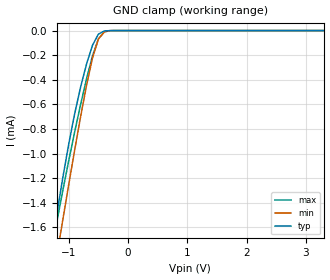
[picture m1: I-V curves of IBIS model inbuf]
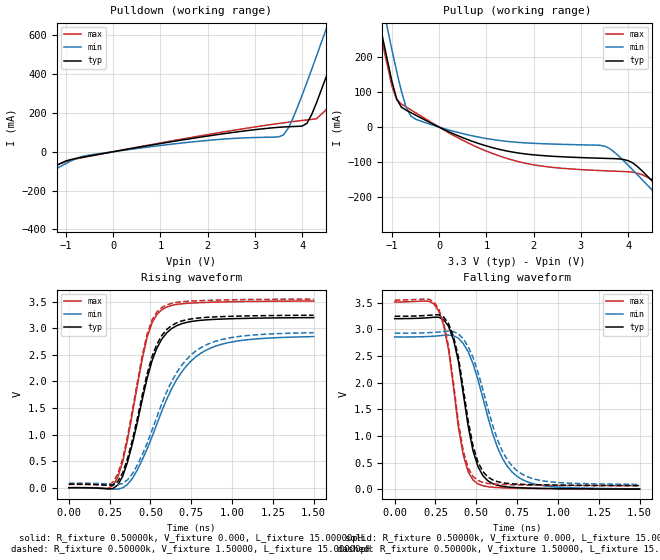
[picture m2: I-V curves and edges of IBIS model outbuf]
| IBIS file 4v38075z.ibs created by s2ibis2 version 1.2
| North Carolina State University Electronics Research Laboratory  1995
[IBIS ver]   3.2
[File name]   4v38075z.ibs
[File Rev]   0.2
[Date]   08/30/2004
[Source]   Integrated Device Technology, Inc.
[Notes]   1.Temperatures: typ=25C, min=150C, max=0C 2.Ramp rates based
   on 500 ohm load.
[Disclaimer] Integrated Device Technology, Inc. ("IDT") hereby grants the
   user of this IBIS model a non-exclusive, nontransferable
   license to use this IBIS model under the following terms. The
   user is granted this license only to use the IBIS model and is
   not granted rights to sell, copy (except as needed to run the
   IBIS model), rent, lease or sub-license the IBIS model in
   whole or in part, or in modified form to anyone. The User may
   modify the IBIS model to suit its specific applications, but
   rights to derivative works and such modifications shall belong
   to IDT. This IBIS model is provided on an AS IS" basis and IDT
   makes absolutely no warranty with respect to the information
   contained herein. IDT DISCLAIMS AND CUSTOMER WAIVES ALL
   WARRANTIES, EXPRESS AND IMPLIED, INCLUDING WARRANTIES OF
   MERCHANTABILITY AND FITNESS FOR A PARTICULAR PURPOSE. THE
   ENTIRE RISK AS TO QUALITY AND PERFORMANCE IS WITH THE USER
   ACCORDINGLY, IN NO EVENT SHALL IDT BE LIABLE FOR ANY DIRECT OR
   INDIRECT DAMAGES, WHETHER IN CONTRACT OR TORT, INCLUDING ANY
   LOST PROFITS OR OTHER INCIDENTAL, CONSEQUENTIAL, EXEMPLARY, OR
   PUNITIVE DAMAGES ARISING OUT OF THE USE OR APPLICATION OF THE
   IBIS model. Further, IDT reserves the right to make changes
   without notice to any product herein to improve reliability,
   function, or design. IDT does not convey any license under
   patent rights or any other intellectual property rights,
   including those of third parties. IDT is not obligated to
   provide maintenance or support for the licensed IBIS model.
[Copyright]   Copyright 1997, Integrated Device Technology, Inc. all rights
   reserved
|   Component idt4v38075z
[Component]   idt4v38075z
[Manufacturer]   Integrated Device Technology, Inc.
[Package]
| variable   typ   min   max
R_pkg   53.14m   52.77m   53.55m
L_pkg   5.18nH   4.04nH   6.38nH
C_pkg   0.38pF   0.224pF   0.551pF
[Pin]  signal_name   model_name   R_pin   L_pin   C_pin
1   O5   outbuf
2   VCC   POWER
3   IN   inbuf
4   GND   GND
5   O1   outbuf
6   O2   outbuf
7   O3   outbuf
8   O4   outbuf
| Models and submodels in the file (2): inbuf (Input), outbuf (Output)
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|   Model inbuf
[Model]   inbuf
Model_type   Input
Polarity   Inverting
Vinl =  0.80000V
Vinh =  2.00000V
Vmeas =  1.50000V
C_comp   2.60000pF   NA   NA
[Temperature Range]   25.00000   0.15000k   0.000
[Voltage Range]   3.30000V   3.00000V   3.60000V
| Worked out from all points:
|   GND clamp passes 1 mA (typ) near -1.03 V on its own axis
[GND_clamp]
| voltage   I(typ)   I(min)   I(max)
-3.3V     -8.354mA   -8.197mA   -8.333mA
-1.3V     -1.792mA   -2.121mA   -1.821mA
-1.2V     -1.488mA   -1.827mA   -1.552mA
-1.1V     -1.195mA   -1.537mA   -1.299mA
-1V       -921.4uA   -1.25mA    -1.056mA
-900mV    -674.9uA   -969.9uA   -823.3uA
-800mV    -458.9uA   -699.2uA   -600.1uA
-700mV    -271.4uA   -445uA     -391uA
-600mV    -119.9uA   -223.2uA   -205.7uA
-500mV    -28.6uA    -68.61uA   -67.73uA
-400mV    -2.904uA   -10.33uA   -9.139uA
3.3V      2.359pA    530.5pA    3.467pA
[POWER_clamp]
| voltage   I(typ)   I(min)   I(max)
-3.3V     0A         0A         0A
-3.2V     0A         0A         0A
-3.1V     0A         0A         0A
0V        0A         0A         0A
|   Model outbuf
[Model]   outbuf
Model_type   Output
Polarity   Non-Inverting
Vmeas =  1.50000V
C_comp   5.50000pF   NA   NA
[Temperature Range]   25.00000   0.15000k   0.000
[Voltage Range]   3.30000V   3.00000V   3.60000V
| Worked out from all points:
|   slope of the pulldown table from 0 to 0.495 V, typ, clamps not added: 23.3 ohm
|   slope of the pullup table from 0 to 0.495 V, typ, clamps not added: 16.5 ohm
|   rising waveform, R_fixture 0.50000k, V_fixture 0.000, L_fixture 15.00000pH: 20-80 % time 158ps typ, 260ps min, 133ps max; typ from 0 V to 3.2 V
|   rising waveform, R_fixture 0.50000k, V_fixture 1.50000, L_fixture 15.00000pH: 20-80 % time 155ps typ, 250ps min, 132ps max; typ from 0.066 V to 3.24 V
|   falling waveform, R_fixture 0.50000k, V_fixture 0.000, L_fixture 15.00000pH: 20-80 % time 110ps typ, 174ps min, 99.2ps max; typ from 3.2 V to 0.004 V
|   falling waveform, R_fixture 0.50000k, V_fixture 1.50000, L_fixture 15.00000pH: 20-80 % time 111ps typ, 178ps min, 99.4ps max; typ from 3.25 V to 0.07 V
[Pulldown]
| voltage   I(typ)   I(min)   I(max)
-3.3V     -367.5mA   -386.3mA   -364.3mA
-1.3V     -81.78mA   -100.8mA   -79.3mA
-700mV    -30.42mA   -27.37mA   -32.6mA
3.5V      125.9mA    76.55mA    145.4mA
3.7V      128.7mA    119.8mA    151.9mA
4V        132.3mA    293.5mA    161mA
4.2V      192.4mA    424.8mA    166.6mA
4.5V      381.8mA    628.3mA    214.5mA
4.9V      655.6mA    904.8mA    470.1mA
5.1V      794.9mA    1.044A     607.7mA
5.3V      935mA      1.184A     746.9mA
6.6V      1.855A     2.106A     1.664A
[Pullup]
| voltage   I(typ)   I(min)   I(max)
-3.3V     1.721A     1.811A     1.704A
-1.3V     322mA      418.1mA    303.8mA
-1V       131.3mA    221.6mA    117.8mA
-900mV    81.55mA    160.2mA    79.28mA
-700mV    48.88mA    57.36mA    57.92mA
-500mV    34.64mA    22.99mA    41.35mA
1.4V      -67.44mA   -40.28mA   -88.17mA
3.5V      -89.46mA   -54.18mA   -125mA
4V        -96.16mA   -109.3mA   -127.8mA
4.5V      -153.5mA   -179.6mA   -150mA
5.3V      -270.5mA   -296mA     -261.5mA
6.6V      -467.1mA   -488.9mA   -460.3mA
[Ramp]
| variable   typ   min   max
dV/dt_r   1.91880/0.15618n   1.70460/0.25896n   2.10600/0.13118n
dV/dt_f   1.89024/0.10805n   1.69356/0.17887n   2.06850/96.26246p
R_load = 0.50000k
[Rising Waveform]
R_fixture = 0.50000k
V_fixture = 0.000
L_fixture = 15.00000pH
| time   V(typ)   V(min)   V(max)
0s        201.6uV    209.1uV    235.1uV
240ps     -21.5mV    -15.14mV   -11.92mV
300ps     49.77mV    -26.85mV   194mV
360ps     483.7mV    63.62mV    904.1mV
480ps     2.058V     730.1mV    2.832V
570ps     2.796V     1.441V     3.347V
690ps     3.082V     2.17V      3.458V
840ps     3.155V     2.584V     3.484V
1.05ns    3.182V     2.766V     3.499V
1.5ns     3.198V     2.841V     3.51V
[Rising Waveform]
R_fixture = 0.50000k
V_fixture = 1.50000
L_fixture = 15.00000pH
| time   V(typ)   V(min)   V(max)
0s        66.3mV     83.71mV    62.47mV
240ps     44.8mV     68.4mV     50.38mV
300ps     116.2mV    57.09mV    255.9mV
360ps     551.1mV    149.1mV    965.1mV
480ps     2.143V     836.8mV    2.889V
510ps     2.466V     1.079V     3.154V
570ps     2.864V     1.581V     3.39V
690ps     3.134V     2.297V     3.496V
840ps     3.203V     2.683V     3.521V
1.5ns     3.243V     2.914V     3.547V
[Falling Waveform]
R_fixture = 0.50000k
V_fixture = 0.000
L_fixture = 15.00000pH
| time   V(typ)   V(min)   V(max)
0s        3.202V     2.858V     3.512V
240ps     3.227V     2.872V     3.48V
300ps     3.184V     2.889V     3.074V
330ps     3.056V     2.894V     2.619V
390ps     2.405V     2.836V     1.172V
420ps     1.793V     2.735V     644mV
510ps     427.6mV    2.058V     101.9mV
630ps     75.61mV    783.2mV    32.56mV
750ps     31.31mV    242.7mV    20.68mV
1.5ns     3.996mV    9.428mV    3.034mV
[Falling Waveform]
R_fixture = 0.50000k
V_fixture = 1.50000
L_fixture = 15.00000pH
| time   V(typ)   V(min)   V(max)
0s        3.247V     2.93V      3.549V
240ps     3.273V     2.943V     3.518V
300ps     3.232V     2.962V     3.119V
330ps     3.108V     2.969V     2.678V
390ps     2.486V     2.917V     1.254V
420ps     1.894V     2.823V     719.4mV
510ps     511mV      2.197V     165.6mV
630ps     143.7mV    927.8mV    94.91mV
750ps     97.78mV    347.2mV    82.92mV
1.5ns     70.06mV    93.03mV    65.22mV
